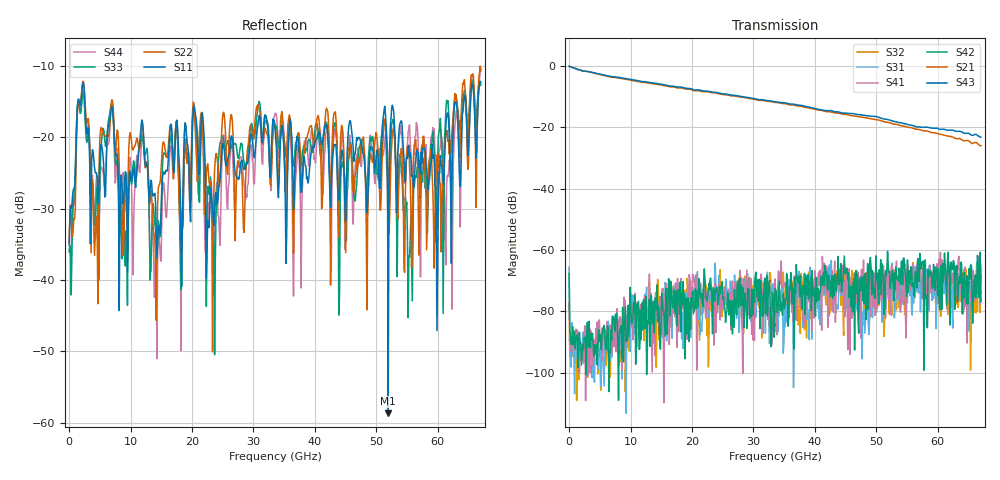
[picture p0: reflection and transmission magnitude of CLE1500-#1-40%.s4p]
!Keysight Technologies,N5247B,US50470101,A.16.20.02
!Date: Thursday, March 13, 2025 10:19:23
!Correction: S11(C  4-Port  )
!S12(C  4-Port  )
!S13(C  4-Port  )
!S14(C  4-Port  )
!S21(C  4-Port  )
!S22(C  4-Port  )
!S23(C  4-Port  )
!S24(C  4-Port  )
!S31(C  4-Port  )
!S32(C  4-Port  )
!S33(C  4-Port  )
!S34(C  4-Port  )
!S41(C  4-Port  )
!S42(C  4-Port  )
!S43(C  4-Port  )
!S44(C  4-Port  )
!S4P File: Measurements: <S11,S12,S13,S14>,
!<S21,S22,S23,S24>,
!<S31,S32,S33,S34>,
!<S41,S42,S43,S44>:
# Hz S  dB  R 50
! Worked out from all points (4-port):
!   601 points, 10 MHz to 67 GHz, reference 50 ohm
!   strongest paths, dB at 10 MHz, 16.76 GHz, 33.51 GHz, 50.25 GHz, 67 GHz:
!     S43: 0.0, -6.5, -11.6, -16.6, -23.2
!     S21: 0.0, -6.7, -11.8, -17.6, -26.0
!     S42: -67.6, -77.5, -72.6, -72.2, -77.0
!     S41: -89.2, -77.0, -69.4, -76.1, -68.1
!     S31: -65.5, -88.8, -81.5, -76.3, -69.9
!     S32: -77.1, -74.9, -86.5, -75.7, -64.9
!   lowest |S11| = -58.7 dB at 51.93 GHz (marker M1), VSWR 1.00, Z = 50.1 - j0.0892 ohm
!   |S11| at or under -10 dB: start of sweep to end of sweep
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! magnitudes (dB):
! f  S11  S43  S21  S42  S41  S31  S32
! 10 MHz  -35.1  0.0  0.0  -67.6  -89.2  -65.5  -77.1
! 2.131 GHz  -13.0  -1.5  -1.6  -93.8  -93.9  -90.4  -95.2
! 4.364 GHz  -25.0  -2.3  -2.4  -93.8  -85.6  -91.4  -88.3
! 14.08 GHz  -29.3  -5.6  -5.9  -75.8  -73.9  -75.7  -76.3
! 20.33 GHz  -15.6  -7.7  -8.0  -79.9  -69.8  -75.5  -79.6
! 51.93 GHz  -58.7  -17.5  -18.4  -65.0  -66.0  -68.3  -64.7
! 67 GHz  -12.3  -23.2  -26.0  -77.0  -68.1  -69.9  -64.9
